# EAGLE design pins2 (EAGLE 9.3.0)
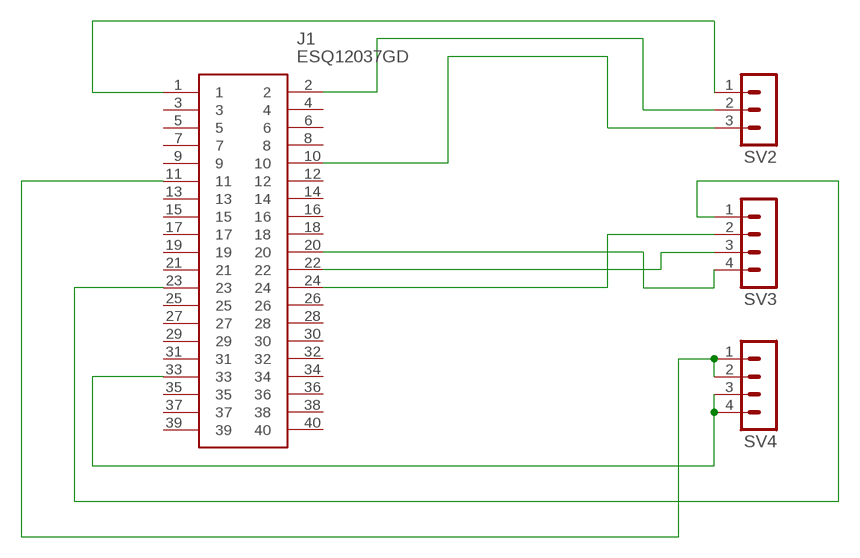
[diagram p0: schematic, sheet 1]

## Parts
J1  ESQ12037GD  [SHDR40W64P254_2X20_5050X495X11]
SV2  MA03-1  [MA03-1]
SV3  MA04-1  [MA04-1]
SV4  MA04-1  [MA04-1]

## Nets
N$1: J1.1 SV2.1
N$2: J1.2 SV2.2
N$3: J1.10 SV2.3
N$4: J1.23 SV3.1
N$5: J1.24 SV3.2
N$6: J1.22 SV3.3
N$7: J1.20 SV3.4
N$8: J1.11 SV4.1 SV4.2
N$9: J1.33 SV4.3 SV4.4
Unconnected: J1.3 J1.4 J1.5 J1.6 J1.7 J1.8 J1.9 J1.12 J1.13 J1.14 J1.15 J1.16 J1.17 J1.18 J1.19 J1.21 J1.25 J1.26 J1.27 J1.28 J1.29 J1.30 J1.31 J1.32 J1.34 J1.35 J1.36 J1.37 J1.38 J1.39 J1.40

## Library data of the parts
J1 = SamacSys_Parts:ESQ12037GD: 2x20 way low insertion short pin PCB skt Samtec 2.54mm 40 Way 2 Row Straight Through Hole Female Multiway Connector Source: Datasheet; DESCRIPTION: 2x20 way low insertion short pin PCB skt Samtec 2.54mm 40 Way 2 Row Straight Through Hole Female Multiway Connector; HEIGHT: 11.3mm; MANUFACTURER_NAME: SAMTEC; MANUFACTURER_PART_NUMBER: ESQ12037GD; RS_PART_NUMBER: 2546182; RS_PRICE-STOCK: http://uk.rs-online.com/web/p/products/2546182
SV2 = con-lstb:MA03-1: PIN HEADER; OC_FARNELL: unknown; OC_NEWARK: unknown
SV3 SV4 = con-lstb:MA04-1: PIN HEADER; OC_FARNELL: unknown; OC_NEWARK: unknown

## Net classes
0 default: width 0.762 mm, drill 0.762 mm, clearance 0.508 mm

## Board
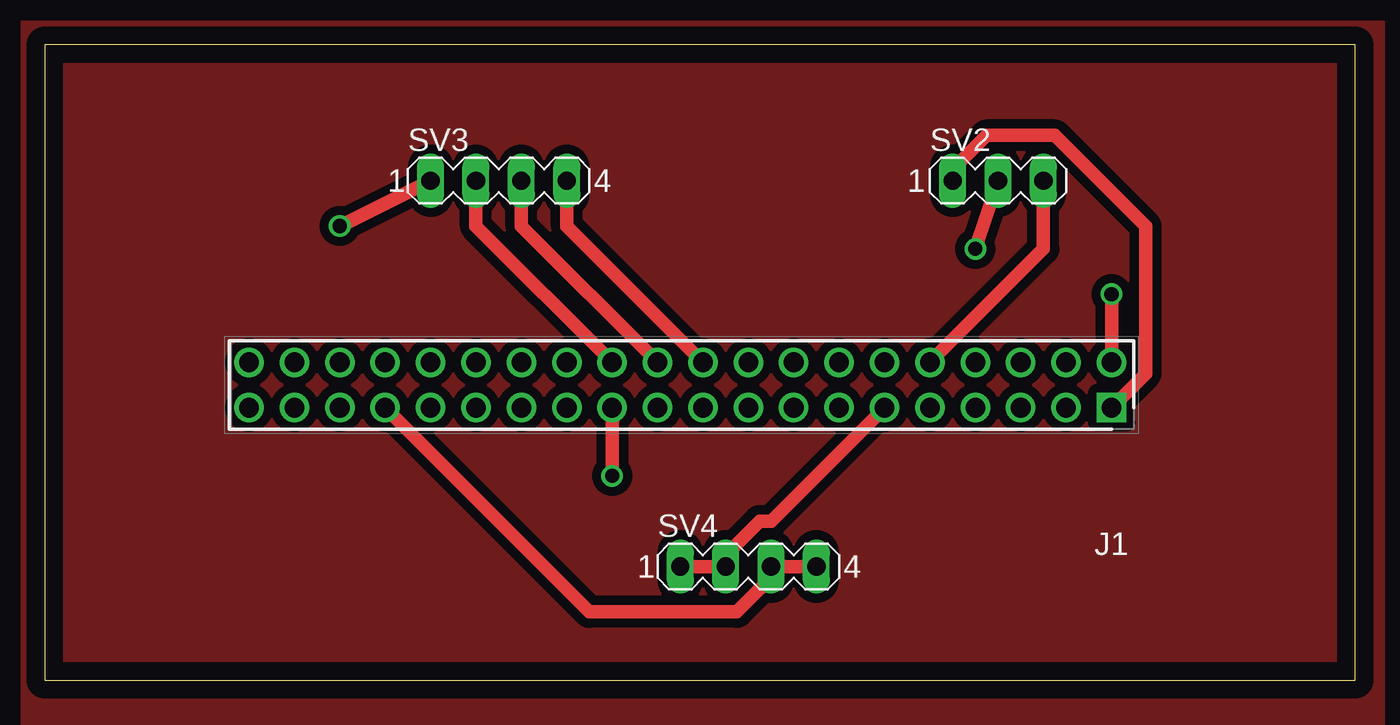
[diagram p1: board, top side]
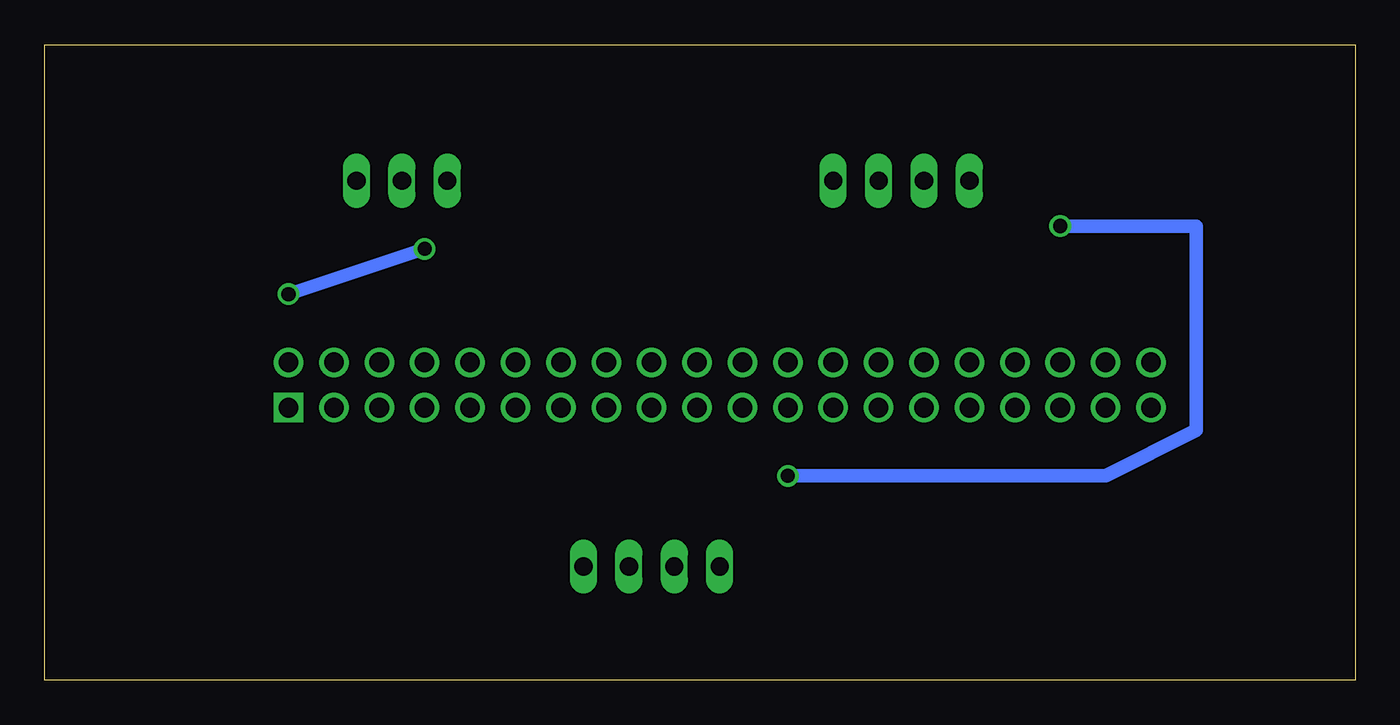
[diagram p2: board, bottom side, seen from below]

Size 73.33 x 35.55 mm. Coordinates in mm from the lower left corner, seen from the top.
Outline: 0,0 73.33,0 73.33,35.55 0,35.55 0,0
Copper layers (1*16): Top 0.035mm / dielectric 1.5mm / Bottom 0.035mm
Design rules "default": minimum track width 6mil, minimum drill 0.35mm, track to track 6mil, track to pad 6mil, pad to pad 6mil, via to via 6mil, smd to smd 6mil, copper to edge 40mil, drill to drill 6mil, minimum pad ring 10mil, minimum via ring 8mil, stop-mask expansion 4mil, vias tented up to drill 0mil, thermal gap 10mil

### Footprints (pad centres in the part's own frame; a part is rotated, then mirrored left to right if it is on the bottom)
SHDR40W64P254_2X20_5050X495X11 = drill 1.1 pad 1.65 square: 1 0,0 | drill 1.1 pad 1.65: 2 0,2.54; 3 -2.54,0; 4 -2.54,2.54; 5 -5.08,0; 6 -5.08,2.54; 7 -7.62,0; 8 -7.62,2.54; 9 -10.16,0; 10 -10.16,2.54; 11 -12.7,0; 12 -12.7,2.54; 13 -15.24,0; 14 -15.24,2.54; 15 -17.78,0; 16 -17.78,2.54; 17 -20.32,0; 18 -20.32,2.54; 19 -22.86,0; 20 -22.86,2.54; 21 -25.4,0; 22 -25.4,2.54; 23 -27.94,0; 24 -27.94,2.54; 25 -30.48,0; 26 -30.48,2.54; 27 -33.02,0; 28 -33.02,2.54; 29 -35.56,0; 30 -35.56,2.54; 31 -38.1,0; 32 -38.1,2.54; 33 -40.64,0; 34 -40.64,2.54; 35 -43.18,0; 36 -43.18,2.54; 37 -45.72,0; 38 -45.72,2.54; 39 -48.26,0; 40 -48.26,2.54
MA03-1 = drill 1.016 long: 1 -2.54,0; 2 0,0; 3 2.54,0
MA04-1 = drill 1.016 long: 1 -3.81,0; 2 -1.27,0; 3 1.27,0; 4 3.81,0

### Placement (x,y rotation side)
J1  59.69,15.24 0 top
SV2  53.34,27.94 0 top
SV3  25.4,27.94 0 top
SV4  39.37,6.35 0 top

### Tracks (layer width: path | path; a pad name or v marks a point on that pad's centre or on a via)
GND
  pour Top: -1.27,36.83 -1.27,-2.54 74.93,-2.54 74.93,36.83
N$1
  Top 0.762: SV2.1 50.8,28.58 52.7,30.48 56.52,30.48 61.59,25.4 61.59,17.15 J1.1
N$2  (via drill 0.8)
  Top 0.762: SV2.2 v52.07,24.13 | J1.2 v59.69,21.59
  Bottom 0.762: v52.07,24.13 v59.69,21.59
N$3
  Top 0.762: SV2.3 55.88,24.13 J1.10
N$4  (via drill 0.8)
  Top 0.762: v16.51,25.4 SV3.1 | J1.23 v31.75,11.43
  Bottom 0.762: v16.51,25.4 8.89,25.4 8.89,13.97 13.97,11.43 v31.75,11.43
N$5
  Top 0.762: SV3.2 24.13,25.4 J1.24
N$6
  Top 0.762: SV3.3 26.67,25.4 J1.22
N$7
  Top 0.762: SV3.4 29.21,25.4 J1.20
N$8
  Top 0.762: 37.47,6.35 SV4.1 | J1.11 40.64,8.89 40,8.89 37.47,6.35 | 37.47,6.35 SV4.2
N$9
  Top 0.762: SV4.4 41.28,6.35 | J1.33 30.48,3.81 38.73,3.81 41.28,6.35 | 41.28,6.35 SV4.3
